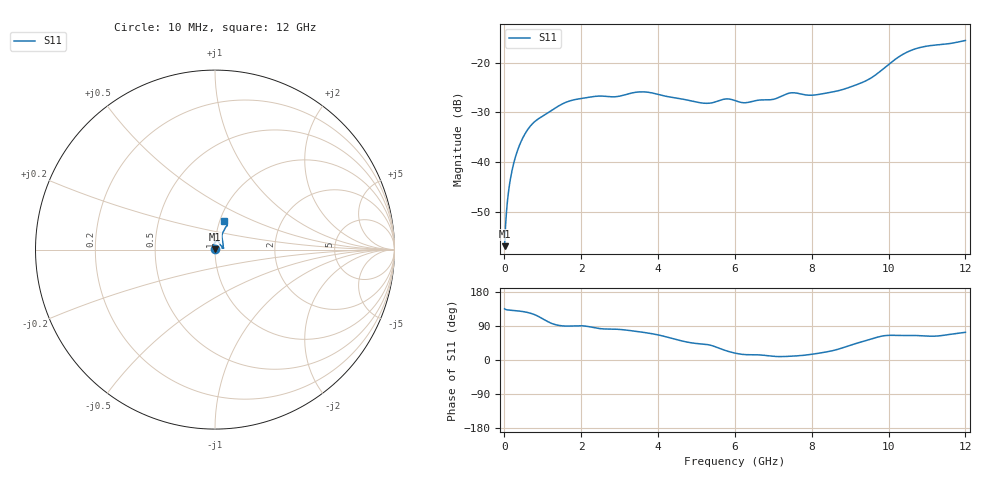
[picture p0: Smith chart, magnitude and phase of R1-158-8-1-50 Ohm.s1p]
!version-1
!date-10.2020
!Series
#GHZ	S	RI	R	50.0
!FREQ.GHZ	S11RE	S11IM
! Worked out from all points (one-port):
!   500 points, 10 MHz to 12 GHz, reference 50 ohm
!   lowest |S11| = -57.0 dB at 10 MHz (marker M1), VSWR 1.00, Z = 49.9 + j0.0998 ohm
!   |S11| at or under -10 dB: start of sweep to end of sweep
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0.01  -0.001 0.001
0.0340281  -0.00155 0.00164
0.0820842  -0.00266 0.00293
0.106112  -0.00321 0.00358
0.178196  -0.00482 0.00551
0.298337  -0.00737 0.00875
0.442505  -0.01 0.0127
0.610701  -0.0122 0.0173
0.778898  -0.0126 0.0218
1.52377  9.75e-06 0.0386
1.8121  -3e-05 0.0422
2.31669  0.00336 0.0454
3.01351  0.00755 0.0455
3.63824  0.0151 0.0485
4.52727  0.0265 0.0348
5.22409  0.0292 0.0259
5.77673  0.0393 0.0178
6.01701  0.0394 0.0127
6.25729  0.0382 0.00976
6.95411  0.0418 0.00744
7.50675  0.049 0.00884
8.08343  0.0454 0.0132
9.02052  0.0441 0.0363
9.54914  0.04 0.0578
10.1979  0.0465 0.0995
10.5103  0.0552 0.1169
10.9187  0.0646 0.1299
12  0.0489 0.1602
